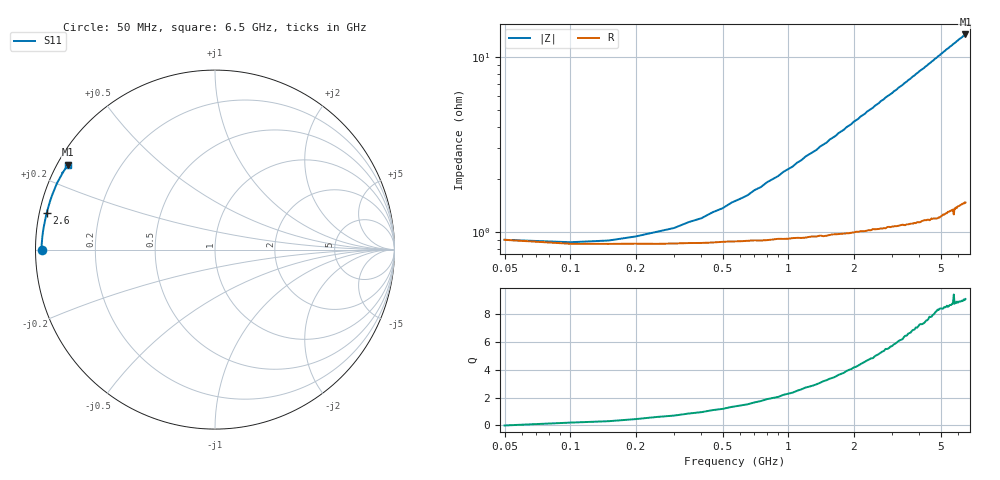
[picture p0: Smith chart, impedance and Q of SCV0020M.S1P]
! Infineon Technologies  Discrete & RF Semiconductors
! BAR63-02L
! Si PIN Diode in TSLP-2
! IF = 20 mA
! S-Parameters:  March  2002
# GHz  S  MA  R  50
!  f  S11
! GHz  MAG  ANG
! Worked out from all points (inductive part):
!   130 points, 50 MHz to 6.5 GHz, reference 50 ohm
!   read as one part to ground: L = 329 pH near 1.4 GHz
!   highest Q = 9.1 at 6.5 GHz (marker M1), where L = 328 pH
!   S11 on the Smith chart (normalised r, x): 50 MHz: 0.02, +0.00; 2.6 GHz: 0.02, +0.11; 6.5 GHz: 0.03, +0.27
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0.05  0.9646 180.0
0.1  0.9664 179.6
0.15  0.9664 179.4
0.25  0.9664 178.8
0.55  0.9654 177.3
0.65  0.9651 176.9
0.8  0.9648 176.1
0.9  0.9642 175.7
1.2  0.9637 174.2
1.35  0.9631 173.6
1.7  0.962 171.9
1.8  0.9618 171.5
2.3  0.9604 169.1
2.45  0.9597 168.5
2.5  0.9599 168.2
2.6  0.9597 167.8
2.8  0.9594 166.8
3  0.9586 166.0
3.2  0.9583 165.0
3.3  0.9579 164.6
4  0.9568 161.3
4.1  0.9561 160.9
4.9  0.9545 157.2
5.7  0.9504 153.5
5.75  0.9535 153.3
5.8  0.9497 153.1
6.05  0.9485 151.9
6.5  0.9466 150.0
